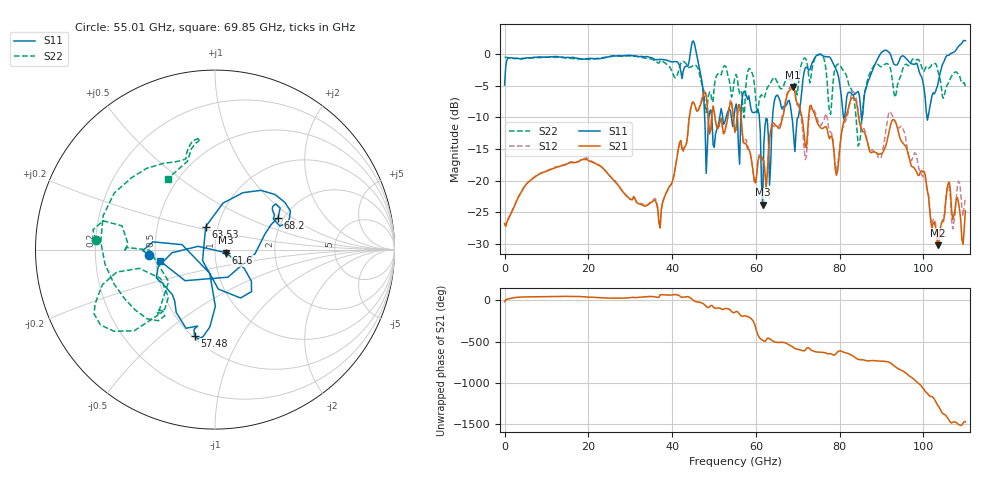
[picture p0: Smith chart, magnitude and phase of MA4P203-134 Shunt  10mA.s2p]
!Keysight Technologies,N5247B,US61255204,A.15.70.20
!Date: Friday, October 21, 2022 15:22:53
!Correction: S11(C  4-Port  )
!S31(C  4-Port  )
!S13(C  4-Port  )
!S33(C  4-Port  )
!S2P File: Measurements: S11, S31, S13, S33:
# Hz S  dB  R 50
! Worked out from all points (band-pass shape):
!   401 points, 10 MHz to 110 GHz, reference 50 ohm
!   highest |S21| = -5.23 dB at 68.75 GHz (marker M1); lowest = -30.2 dB at 103.4 GHz (marker M2)
!   |S21| within 3 dB of the highest: 66.92 GHz to 70.34 GHz (3.428 GHz wide, 4.99 % of centre); 82.18 GHz to 84.16 GHz (1.976 GHz wide, 2.38 % of centre)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
!   lowest |S11| = -23.8 dB at 61.6 GHz (marker M3), VSWR 1.14, Z = 56.6 - j1.98 ohm
!   |S11| at or under -10 dB: 49.44 GHz to 51.36 GHz (1.917 GHz wide, 3.8 % of centre); 60.82 GHz to 63.98 GHz (3.16 GHz wide, 5.06 % of centre); 68.6 GHz to 70.13 GHz (1.526 GHz wide, 2.2 % of centre)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
!   |S22| runs from -14.5 to 0.0 dB; largest |S21 - S12| = 0.17
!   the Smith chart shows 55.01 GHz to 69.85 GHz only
!   S11 on the Smith chart (normalised r, x): 55.01 GHz: 0.46, -0.03; 57.48 GHz: 0.51, -0.65; 61.6 GHz: 1.13, -0.04; 63.53 GHz: 0.87, +0.23; 68.2 GHz: 1.87, +0.79; 69.85 GHz: 0.53, -0.08
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1e7  -4.93 -179.2  -26.76 -14.3  -26.75 -14.3  -0.60 -179.4
1.843332e10  -0.85 145.7  -16.70 45.5  -16.67 45.3  -0.80 145.3
3.685665e10  -0.90 154.6  -26.70 39.1  -26.37 39.6  -1.45 154.2
4.51059e10  2.02 85.1  -7.66 -0.5  -7.62 -2.6  -1.76 115.3
4.813062e10  -18.84 60.1  -6.58 -71.5  -6.41 -72.0  -9.25 113.3
5.5005e10  -8.61 -175.8  -12.29 -142.5  -12.54 -144.1  -3.52 175.6
5.747978e10  -6.12 -103.4  -14.10 172.7  -13.48 178.0  -6.26 -131.2
6.16044e10  -23.80 -15.7  -16.56 -122.8  -16.66 -120.7  -6.75 -132.9
6.352922e10  -17.18 111.9  -12.03 -113.5  -12.41 -110.4  -4.52 -161.2
6.82038e10  -8.09 27.0  -5.66 173.5  -5.20 170.4  -4.02 98.2
6.875375e10  -10.76 17.0  -5.23 157.8  -4.96 153.9  -4.26 98.5
6.985365e10  -10.15 -167.9  -7.84 131.3  -8.12 130.8  -6.47 123.6
7.342832e10  -1.37 178.2  -8.69 112.1  -8.67 107.5  -2.24 156.3
7.645305e10  -0.44 -165.6  -11.53 87.1  -9.92 118.8  -1.30 148.0
7.947778e10  -3.02 -147.6  -18.54 96.5  -17.73 95.0  -1.66 -137.2
8.415235e10  -6.05 -39.1  -8.21 12.9  -7.75 17.7  -12.30 -170.4
8.745205e10  -3.21 49.8  -15.59 -8.4  -15.21 5.1  -2.70 53.5
9.185165e10  0.20 88.6  -12.05 -30.5  -9.09 -23.1  -1.92 76.1
9.817608e10  -1.49 176.0  -18.39 104.8  -15.72 103.9  -0.95 -174.5
1.034006e11  -4.91 -37.5  -30.16 169.7  -30.32 173.0  -2.59 -110.8
1.069753e11  0.16 10.4  -26.15 -33.9  -27.61 -37.2  -3.30 -23.4
1.1e11  2.08 46.2  -24.73 -29.2  -22.58 -28.2  -5.19 10.5
